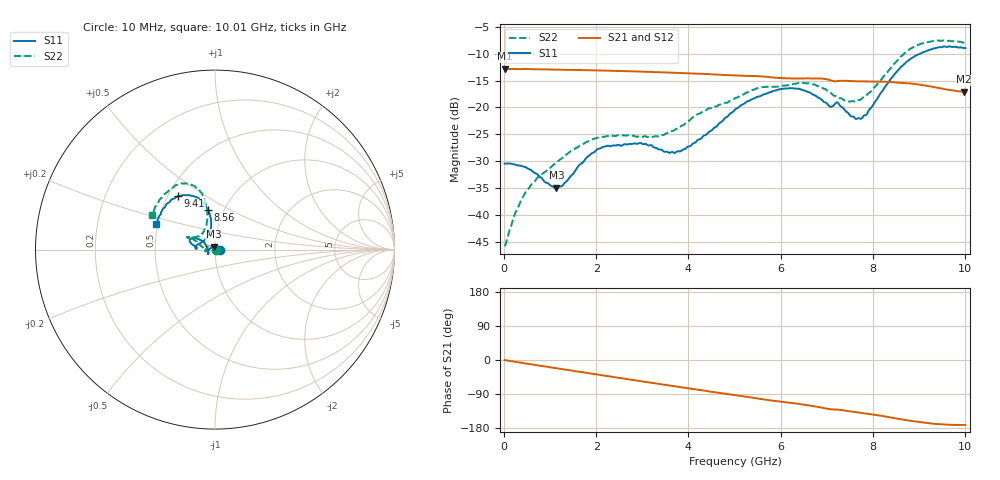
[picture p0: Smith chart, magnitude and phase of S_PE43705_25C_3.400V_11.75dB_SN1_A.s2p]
! Device ID: PE43705
! Serial: 1
! Insertion: A
! Impedance: 50 ohm
! Temp: 25C
! VDD: 3.400V
! Attenuation Step: 11.75dB
#  Hz  S  RI  R  50
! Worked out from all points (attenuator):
!   401 points, 10 MHz to 10.01 GHz, reference 50 ohm
!   highest |S21| = -12.79 dB at 10 MHz (marker M1); lowest = -17.1 dB at 9.985 GHz (marker M2)
!   lowest |S11| = -34.9 dB at 1.135 GHz (marker M3), VSWR 1.04, Z = 49.4 + j1.67 ohm
!   |S11| at or under -10 dB: start of sweep to 9.023 GHz
!   |S22| runs from -45.8 to -7.5 dB; largest |S21 - S12| = 0.0022
!   S11 on the Smith chart (normalised r, x): 10 MHz: 1.06, +0.00; 8.56 GHz: 0.84, +0.39; 9.41 GHz: 0.56, +0.38; 10.01 GHz: 0.49, +0.16
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1e7  0.03 0.000234  0.2293 -0.00109  0.2294 -0.000915  0.00509 0.000362
2.35e8  0.0284 0.00781  0.2272 -0.0186  0.2272 -0.0186  0.00482 0.00903
4.6e8  0.0235 0.015  0.2249 -0.0357  0.2249 -0.0353  0.000946 0.0161
1.135e9  -0.00582 0.0169  0.2088 -0.0832  0.209 -0.0831  -0.0239 0.0187
1.685e9  -0.0301 0.0023  0.1888 -0.1182  0.1889 -0.1181  -0.0447 0.00739
2.21e9  -0.0407 -0.0155  0.1642 -0.1469  0.1643 -0.1469  -0.0536 -0.00572
2.96e9  -0.0398 -0.0246  0.1212 -0.1786  0.1214 -0.1785  -0.0531 -0.00645
3.36e9  -0.0359 -0.0189  0.0961 -0.1899  0.0963 -0.1896  -0.0539 -0.003
3.885e9  -0.0404 0.00218  0.0621 -0.1992  0.0623 -0.199  -0.0672 0.0115
5.01e9  -0.0791 0.0535  -0.00937 -0.1985  -0.00911 -0.1986  -0.1109 0.0503
5.51e9  -0.1096 0.0625  -0.0394 -0.1913  -0.0392 -0.1913  -0.1357 0.0666
5.985e9  -0.1347 0.0612  -0.0633 -0.1769  -0.0622 -0.177  -0.1409 0.0693
6.685e9  -0.1296 0.0311  -0.0969 -0.1589  -0.0968 -0.1589  -0.1487 0.0687
7.41e9  -0.0858 0.0343  -0.1227 -0.1276  -0.1222 -0.128  -0.0859 0.0785
7.71e9  -0.0524 0.0595  -0.132 -0.1152  -0.1315 -0.1153  -0.0644 0.0979
7.91e9  -0.0328 0.0874  -0.1379 -0.1067  -0.1378 -0.1076  -0.0528 0.1252
8.36e9  -0.0235 0.1753  -0.151 -0.0839  -0.1504 -0.0843  -0.0453 0.2216
8.56e9  -0.0385 0.2213  -0.1551 -0.0709  -0.1542 -0.0718  -0.056 0.2776
8.935e9  -0.0942 0.2897  -0.1574 -0.0501  -0.1562 -0.0492  -0.1191 0.3571
9.41e9  -0.2066 0.2971  -0.1499 -0.0287  -0.1494 -0.0287  -0.2192 0.3587
9.985e9  -0.3219 0.151  -0.1387 -0.0211  -0.1391 -0.0217  -0.3439 0.2057
1.001e10  -0.3286 0.1418  -0.1392 -0.0215  -0.1401 -0.0218  -0.3517 0.1944
